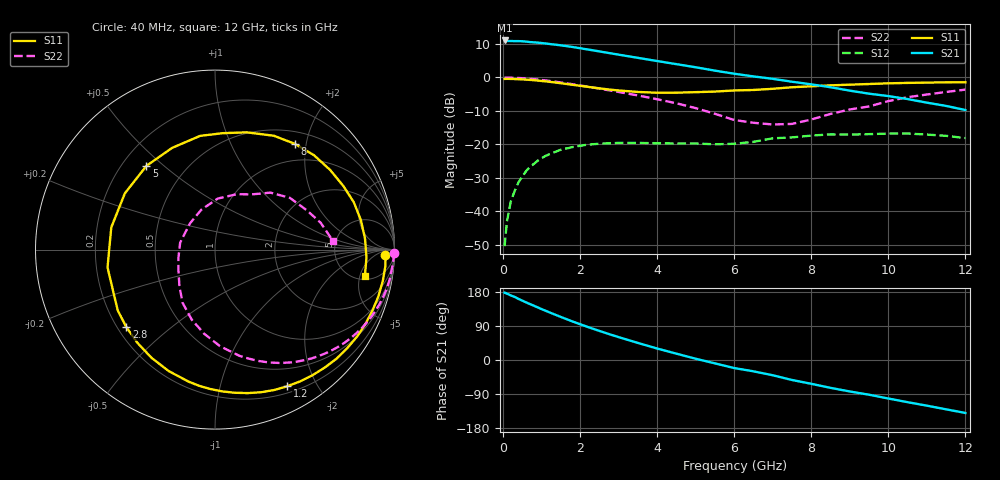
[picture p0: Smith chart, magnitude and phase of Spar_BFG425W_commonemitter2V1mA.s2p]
! Filename: 21bfg425.001
! BFG425W Field C1
! V1=7.884E-001V,V2=2.000E+000V, I1=1.297E-005A, I2=1.000E-003A
# GHz  S  MA  R 50
!  S11  S21  S12  S22
!Freq(GHz)  Mag  Ang  Mag  Ang  Mag  Ang  Mag  Ang
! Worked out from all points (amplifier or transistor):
!   44 points, 40 MHz to 12 GHz, reference 50 ohm
!   highest |S21| = 11.1 dB at 40 MHz (marker M1)
!   |S21| within 3 dB of that: start of sweep to 2.358 GHz
!   unconditionally stable (mu >= 1): 3.42 GHz to end of sweep
!   at 700 MHz: K = 0.13, MSG = 18.7 dB, |S12| = -26.7 dB
!   at 2.4 GHz: K = 0.57, MSG = 14.0 dB, |S12| = -19.9 dB
!   at 12 GHz: K = 2.19, MAG = -2.0 dB, |S12| = -18.1 dB
!   lowest NFmin = 0.70 dB at 900 GHz
!   S11 on the Smith chart (normalised r, x): 40 MHz: 27, -18; 1.2 GHz: 0.28, -1.62; 2.8 GHz: 0.24, -0.36; 5 GHz: 0.30, +0.44; 8 GHz: 0.69, +1.79; 12 GHz: 5.76, -6.03
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0.04  0.95 -1.9  3.575 177.7  0.003 83.5  0.996 -1.1
0.1  0.954 -5.3  3.518 175.2  0.007 87.1  0.996 -3.1
0.2  0.951 -10.5  3.504 170.4  0.014 82.3  0.991 -6.3
0.4  0.941 -21.0  3.493 161.2  0.027 75.1  0.982 -12.6
0.8  0.91 -41.9  3.35 143.2  0.051 60.4  0.943 -24.6
1  0.886 -52.2  3.272 134.3  0.062 53.5  0.916 -30.4
1.2  0.861 -62.2  3.171 125.8  0.071 47.0  0.888 -35.9
1.4  0.835 -72.2  3.072 117.7  0.079 40.6  0.857 -41.2
1.7  0.791 -87.1  2.917 105.7  0.088 31.9  0.809 -48.6
2.2  0.724 -110.9  2.619 87.1  0.099 19.0  0.728 -60.2
2.8  0.656 -138.9  2.292 66.8  0.104 6.4  0.635 -72.9
3.5  0.607 -170.6  1.965 45.0  0.105 -4.9  0.538 -87.2
4  0.591 167.9  1.76 30.3  0.104 -11.1  0.472 -97.4
4.5  0.592 148.0  1.581 16.7  0.103 -15.6  0.411 -108.4
5  0.603 129.3  1.42 3.3  0.103 -20.8  0.348 -121.1
6  0.639 97.5  1.136 -21.3  0.102 -28.5  0.231 -152.1
6.5  0.65 86.3  1.036 -29.9  0.109 -22.7  0.21 -166.5
7.5  0.714 62.6  0.863 -52.8  0.127 -37.4  0.202 133.7
8  0.738 53.1  0.789 -62.8  0.135 -42.9  0.235 109.0
8.5  0.762 43.6  0.714 -73.5  0.141 -51.2  0.285 86.8
10.5  0.829 11.5  0.475 -111.3  0.145 -84.1  0.507 34.7
12  0.848 -10.0  0.326 -139.8  0.124 -115.2  0.658 4.3
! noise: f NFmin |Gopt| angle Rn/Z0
900  0.7  0.67  19.1  0.4
2000  1.3  0.56  57.5  0.36
